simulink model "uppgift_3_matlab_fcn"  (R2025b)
settings: Solver=VariableStepAuto  StartTime=0.0  StopTime=10.0  RelTol=1e-3
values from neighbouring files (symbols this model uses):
  m_dot_end = 14*1e-3    (= 0.014)    [Lektion_2.m]
  m_dot_start = 12*1e-3    (= 0.012)    [Lektion_2.m]
  R = 280    [Lektion_2.m]
  T_i = 320    [Lektion_2.m]
  V_i = 2/1e3    (= 0.002)    [Lektion_2.m]
undefined symbols (not defined in the file or in its folder): p_im

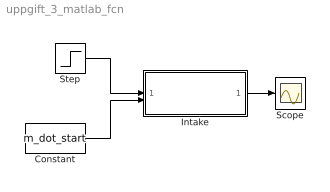
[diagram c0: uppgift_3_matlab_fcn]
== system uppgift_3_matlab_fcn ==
  Constant : Constant  Value=m_dot_start
  Intake : Subsystem
  Scope : Scope
  Step : Step  Time=3  Before=m_dot_start  After=m_dot_end  SampleTime=0
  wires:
  Intake/1(p_im [Pa]) -> Scope/1
  Constant/1 -> Intake/2(m_ac [kg/s])
  Step/1 -> Intake/1(m_at [kg/s])

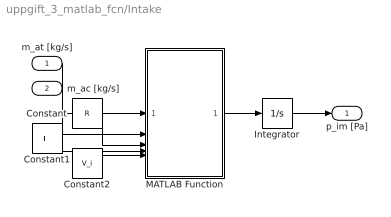
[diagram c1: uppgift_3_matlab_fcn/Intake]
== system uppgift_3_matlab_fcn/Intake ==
  m_at [kg/s] : Inport
  m_ac [kg/s] : Inport  Port=2
  Constant : Constant  Value=R
  Constant1 : Constant  Value=T_i
  Constant2 : Constant  Value=V_i
  Integrator : Integrator  InitialCondition=p_im
  MATLAB Function : MATLAB Function  TreatAsAtomicUnit=on
  p_im [Pa] : Outport
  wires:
  Integrator/1 -> p_im [Pa]/1
  MATLAB Function/1(y) -> Integrator/1
  m_ac [kg/s]/1 -> MATLAB Function/2(m_ac)
  m_at [kg/s]/1 -> MATLAB Function/1(m_at)
  Constant/1 -> MATLAB Function/3(R)
  Constant1/1 -> MATLAB Function/4(T)
  Constant2/1 -> MATLAB Function/5(V)

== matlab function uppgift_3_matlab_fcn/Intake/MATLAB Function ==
function y = fcn(m_at,m_ac,R,T,V)

y = u;
